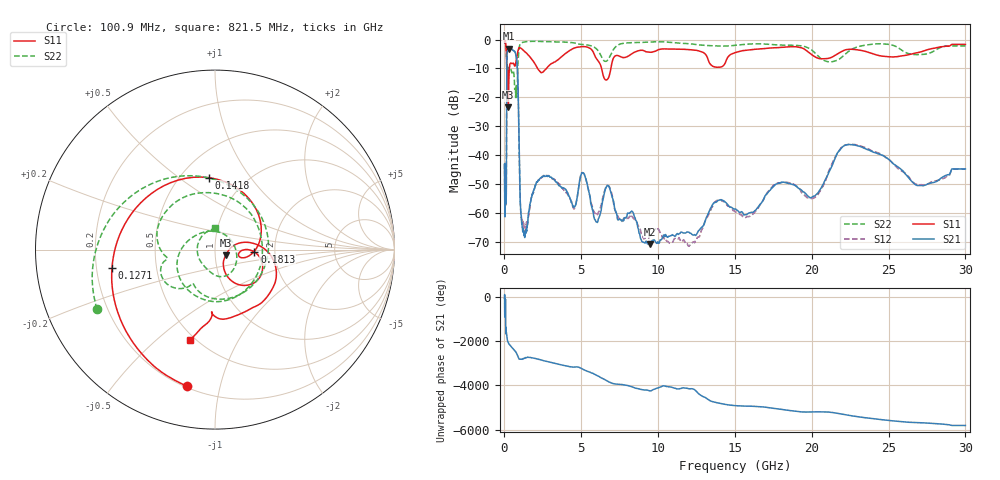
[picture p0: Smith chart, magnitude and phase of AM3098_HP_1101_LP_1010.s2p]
! Date/Time: Thu, Feb 28, 2019 8:45 AM
! Network Analyzer: Agilent Technologies E8364B Rev: A.07.50.67
! Sweep from 0.010 to 30.000 GHz, 1601 Points, Sweep Type: LOG
! Power Supply: 5.022 V, 0.002 A
# Hz S DB R 50
!freq MagS11 AngS11 MagS21 AngS21 MagS12 AngS12 MagS22 AngS22
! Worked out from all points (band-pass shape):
!   1601 points, 10 MHz to 30 GHz, reference 50 ohm
!   highest |S21| = -3.09 dB at 267.8 MHz (marker M1); lowest = -70.7 dB at 9.49 GHz (marker M2)
!   |S21| within 3 dB of the highest: 159.3 MHz to 771.8 MHz (612.5 MHz wide, 132 % of centre)
!   lowest |S11| = -23.4 dB at 252.2 MHz (marker M3), VSWR 1.15, Z = 56.3 - j3.54 ohm
!   |S11| at or under -10 dB: 148 MHz to 319.9 MHz (171.9 MHz wide, 73.5 % of centre); 2.155 GHz to 2.735 GHz (579.3 MHz wide, 23.7 % of centre); 6.321 GHz to 6.925 GHz (604 MHz wide, 9.12 % of centre)
!   |S22| runs from -20.1 to -0.6 dB; largest |S21 - S12| = 0.013
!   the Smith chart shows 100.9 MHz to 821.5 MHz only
!   S11 on the Smith chart (normalised r, x): 100.9 MHz: 0.21, -0.79; 127.1 MHz: 0.27, -0.08; 141.8 MHz: 0.68, +0.65; 181.3 MHz: 1.56, -0.04; 821.5 MHz: 0.47, -0.65
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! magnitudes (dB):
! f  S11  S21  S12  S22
! 10 MHz  -0.4  -44.7  -45.2  -0.6
! 38.04 MHz  -0.3  -57.0  -59.3  -0.8
! 100.9 MHz  -2.2  -56.3  -54.5  -2.7
! 127.1 MHz  -4.7  -42.9  -42.6  -6.0
! 141.8 MHz  -7.9  -17.7  -17.7  -10.5
! 144.7 MHz  -8.8  -14.3  -14.2  -10.7
! 181.3 MHz  -13.1  -4.2  -4.2  -10.9
! 252.2 MHz  -23.4  -3.2  -3.1  -11.4
! 267.8 MHz  -19.1  -3.1  -3.1  -11.3
! 550.5 MHz  -8.2  -3.7  -3.7  -10.8
! 821.5 MHz  -5.6  -8.5  -8.5  -18.5
! 1.029 GHz  -2.9  -56.3  -56.2  -1.6
! 1.154 GHz  -3.3  -64.9  -62.5  -1.0
! 2.084 GHz  -9.3  -49.3  -49.4  -0.6
! 4.503 GHz  -3.0  -58.0  -58.5  -1.1
! 5.128 GHz  -2.4  -46.2  -46.2  -1.7
! 5.929 GHz  -6.1  -62.6  -60.2  -2.9
! 7.926 GHz  -6.1  -61.4  -61.9  -1.2
! 9.49 GHz  -4.4  -70.7  -67.8  -0.9
! 20 GHz  -5.2  -54.5  -55.0  -3.6
! 22.56 GHz  -3.3  -36.3  -36.2  -3.5
! 30 GHz  -1.7  -44.8  -44.8  -2.2
